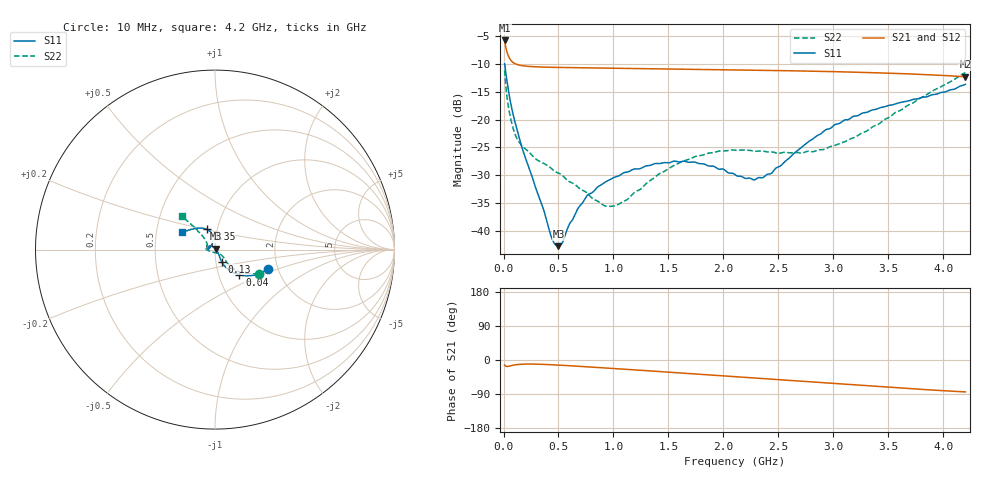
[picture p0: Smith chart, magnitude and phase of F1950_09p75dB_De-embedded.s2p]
! Integrated Device Technology
! Corporate Headquarters
! 6024 Silver Creek Valley Road
! San Jose, CA 95138  USA
! Phone:  1-408-284-8200
! Toll Free:  1-800-223-1366
! Webpage:  http://www.idt.com/
! Timing and RF Division
! 515 Groton Road, Suite 102
! Westford, MA 01886-6024
! Device:  F1950
! Description: 7-bit 0.25 dB Digital Step Attenuator
! Frequency:  150.0 -  4000.00 MHz
! Package:  4x4 mm Thin QFN Plastic Package: 24 pin
! Ports:  2 RF, 12 DC
!  Pin  1  = D0
!  Pin  2  = VDD
!  Pin  3  = Vmode
!  Pin  4  = GND
!  Pin  5  = RF1  =  Port 1
!  Pin  6  = GND
!  Pin  7  = GND
!  Pin  8  = GND
!  Pin  9  = GND
!  Pin 10  = GND
!  Pin 11  = GND
!  Pin 12  = GND
!  Pin 13  = GND
!  Pin 14  = RF2  =  Port 2
!  Pin 15  = GND
!  Pin 16  = LE
!  Pin 17  = CLK
!  Pin 18  = DATE
!  Pin 19  = D6
!  Pin 20  = D5
!  Pin 21  = D4
!  Pin 22  = D3
!  Pin 23  = D2
!  Pin 24  = D1
! State:  39
! Atten State:  9.75 dB
! Voltage:  +5.00 Volts
! Current:  Not Measured mA
! Data:  The device was measured on a the F195X evaluation board which has
!  individual transmission lines to the RF pins.  Data was collected
!  using a calibrated network analyzer.  The evaluation board was
!  de-embedded using a TRL calibration technique.
!  The reference plane is the edge of the package pin.
! Misc:  Board 2019
!  Action Tracker AT0250
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# GHz S dB R 50
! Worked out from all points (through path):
!   420 points, 10 MHz to 4.2 GHz, reference 50 ohm
!   highest |S21| = -5.75 dB at 10 MHz (marker M1); lowest = -12.3 dB at 4.2 GHz (marker M2)
!   group delay of S21, straight-line fit = 52.5 ps
!   lowest |S11| = -42.8 dB at 500 MHz (marker M3), VSWR 1.01, Z = 50.5 + j0.533 ohm
!   |S11| at or under -10 dB: 10.25 MHz to end of sweep
!   |S22| runs from -35.6 to -11.1 dB; largest |S21 - S12| = 0.00038
!   S11 on the Smith chart (normalised r, x): 10 MHz: 1.78, -0.43; 40 MHz: 1.26, -0.37; 130 MHz: 1.07, -0.14; 3.35 GHz: 0.89, +0.20; 4.2 GHz: 0.68, +0.14
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0.01  -9.96 -20.2  -5.75 -13.4  -5.75 -13.4  -11.12 -29.3
0.04  -14.17 -45.9  -8.34 -16.9  -8.34 -16.9  -17.11 -47.1
0.08  -18.44 -58.2  -9.60 -14.2  -9.60 -14.2  -21.05 -46.2
0.13  -22.35 -61.3  -10.12 -11.8  -10.12 -11.8  -23.69 -41.9
0.29  -32.15 -47.9  -10.49 -10.8  -10.49 -10.9  -27.04 -39.9
0.44  -41.40 -0.8  -10.59 -12.6  -10.58 -12.6  -28.90 -41.2
0.5  -42.79 46.7  -10.61 -13.5  -10.61 -13.5  -29.63 -44.3
0.53  -42.36 64.8  -10.62 -13.9  -10.62 -13.9  -29.96 -44.4
0.6  -38.80 95.8  -10.64 -15.1  -10.64 -15.1  -31.20 -48.6
0.71  -35.20 114.8  -10.67 -17.0  -10.67 -17.1  -32.64 -57.4
0.91  -31.46 133.6  -10.73 -20.7  -10.72 -20.8  -35.42 -86.8
1  -30.46 139.6  -10.75 -22.4  -10.75 -22.4  -35.57 -108.0
1.41  -27.92 164.6  -10.85 -30.3  -10.85 -30.3  -29.83 -164.8
1.73  -27.64 174.5  -10.94 -36.5  -10.94 -36.5  -26.77 -179.4
2.11  -29.98 165.3  -11.05 -44.1  -11.05 -44.1  -25.53 170.2
2.27  -30.83 145.6  -11.10 -47.3  -11.10 -47.3  -25.64 166.3
2.36  -30.43 132.3  -11.13 -49.0  -11.13 -49.1  -25.66 163.9
2.81  -23.53 100.1  -11.29 -58.1  -11.29 -58.1  -25.78 147.1
3.09  -20.18 103.6  -11.41 -63.7  -11.41 -63.8  -24.08 139.2
3.35  -18.28 112.2  -11.55 -68.9  -11.55 -69.0  -21.38 133.8
3.51  -17.42 118.2  -11.65 -72.0  -11.64 -72.1  -19.58 132.7
4.2  -13.65 151.3  -12.30 -84.2  -12.29 -84.3  -11.53 134.7
